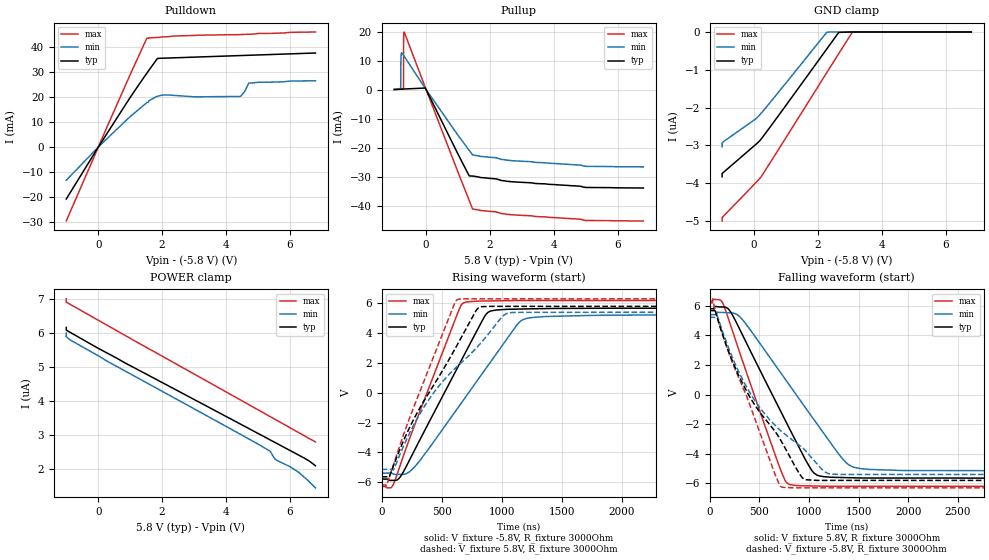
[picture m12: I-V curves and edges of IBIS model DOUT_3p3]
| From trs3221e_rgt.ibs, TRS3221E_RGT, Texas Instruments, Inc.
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[Model]   DOUT_3p3
Model_type   3-state
Polarity   Inverting
Vmeas = 1.65
Vref = 0
Cref = 150pF
Rref = 3000
|variable   typ   min   max
C_comp   6.67pF   5.86pF   7.62pF
|C_pullup   6.73pF   5.94pF   7.44pF
|C_pulldown   6.54pF   5.54pF   7.65pF
[Voltage Range]   11.6   10.8   12.6
[Temperature Range]   27   110   -40
[Pullup Reference]   5.8   5.4   6.3
[Pulldown Reference]   -5.8   -5.4   -6.3
[Power Clamp Reference]   5.8   5.4   6.3
[GND Clamp Reference]   -5.8   -5.4   -6.3
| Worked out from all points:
|   slope of the pulldown table from 0 to 1.74 V, typ, clamps not added: 52 ohm
|   slope of the pullup table from 0 to 1.74 V, typ, clamps not added: 57.4 ohm
|   falling waveform, V_fixture 5.8V, R_fixture 3000Ohm: 20-80 % time 516ns typ, 670ns min, 385ns max; typ from 5.8 V to -5.64 V
|   rising waveform, V_fixture -5.8V, R_fixture 3000Ohm: 20-80 % time 446ns typ, 563ns min, 354ns max; typ from -5.8 V to 5.67 V
|   rising waveform, V_fixture 5.8V, R_fixture 3000Ohm: 20-80 % time 475ns typ, 608ns min, 355ns max; typ from -5.64 V to 5.8 V
|   falling waveform, V_fixture -5.8V, R_fixture 3000Ohm: 20-80 % time 586ns typ, 680ns min, 425ns max; typ from 5.67 V to -5.8 V
[Pulldown]
|   Voltage   I(typ)   I(min)   I(max)
-1V       -20.69mA   -13.21mA   -29.48mA
121.7mV   2.419mA    1.551mA    3.562mA
975.3mV   19.36mA    11.94mA    28.26mA
1.525V    29.58mA    17.81mA    43.51mA
1.856V    35.45mA    20.31mA    43.81mA
2.156V    35.58mA    20.85mA    44.08mA
3.033V    35.96mA    20.07mA    44.64mA
4.428V    36.57mA    20.23mA    44.94mA
4.464V    36.58mA    20.4mA     44.96mA
4.586V    36.64mA    22.27mA    45.02mA
4.713V    36.69mA    25.62mA    45.08mA
6.8V      37.6mA     26.51mA    45.97mA
[GND Clamp]
|   Voltage   I(typ)   I(min)   I(max)
-1V       -3.829uA   -3.033uA   -4.999uA
-1V       -3.77uA    -2.976uA   -4.939uA
-1V       -3.759uA   -2.965uA   -4.928uA
-1V       -3.742uA   -2.949uA   -4.912uA
-999.7mV  -3.742uA   -2.934uA   -4.909uA
-947.7mV  -3.704uA   -2.894uA   -4.86uA
29.67mV   -2.991uA   -2.31uA    -4.007uA
240.5mV   -2.811uA   -2.129uA   -3.804uA
2.272V    -452.5nA   -9.865nA   -1.078uA
2.65V     -10.91nA   0A         -571.9nA
3.071V    0A         0A         -11.58nA
6.8V      0A         0A         0A
[Pullup]
|   Voltage   I(typ)   I(min)   I(max)
-1V       58.5uA     47.9uA     71.7uA
-800mV    163.2uA    219.8uA    162.4uA
-787.3mV  169.9uA    11.17mA    168.1uA
-778.7mV  174.4uA    12.51mA    172.1uA
-709.6mV  210.6uA    11.87mA    203.4uA
-706.5mV  212.2uA    11.82mA    1.796mA
-705.2mV  212.9uA    11.8mA     14.41mA
-703.4mV  213.9uA    11.77mA    18.21mA
-686.7mV  222.6uA    11.49mA    19.85mA
-24.92mV  569.4uA    410.9uA    731.3uA
1.455V    -29.77mA   -22.5mA    -41.14mA
6.8V      -33.87mA   -26.6mA    -45.24mA
[POWER Clamp]
|   Voltage   I(typ)   I(min)   I(max)
-1V       6.156uA    5.99uA     6.993uA
-1V       6.096uA    5.932uA    6.931uA
-1V       6.077uA    5.912uA    6.913uA
-999.8mV  6.077uA    5.883uA    6.897uA
-868.1mV  6.007uA    5.785uA    6.827uA
970.8mV   5.052uA    4.814uA    5.854uA
5.366V    2.871uA    2.54uA     3.554uA
5.514V    2.798uA    2.325uA    3.476uA
5.566V    2.772uA    2.277uA    3.449uA
6V        2.555uA    2.08uA     3.221uA
6.25V     2.431uA    1.93uA     3.09uA
6.8V      2.106uA    1.459uA    2.802uA
[Ramp]
R_load = 3000
|   typ   min   max
dV/dt_r   6.88152/4.46257e-07   6.37012/5.61965e-07   7.49789/3.54595e-07
dV/dt_f   6.86701/5.15292e-07   6.32828/6.69404e-07   7.49815/3.85293e-07
[Falling Waveform]
V_fixture = 5.8V
V_fixture_min = 5.4V
V_fixture_max = 6.3V
R_fixture = 3000Ohm
C_fixture = 0F
|   Time   V(typ)   V(min)   V(max)
0s        5.8V       5.4V       6.3V
136.4ns   5.912V     5.54V      6.107V
209.2ns   5.601V     5.519V     4.713V
317.9ns   4.199V     5.153V     2.525V
693.4ns   -842.9mV   1.677V     -4.712V
794.9ns   -2.189V    714.4mV    -6.045V
1.051us   -5.31V     -1.711V    -6.174V
1.327us   -5.601V    -4.254V    -6.191V
1.469us   -5.625V    -4.937V    -6.191V
4us       -5.645V    -5.148V    -6.197V
[Rising Waveform]
V_fixture = -5.8V
V_fixture_min = -5.4V
V_fixture_max = -6.3V
R_fixture = 3000Ohm
C_fixture = 0F
|   Time   V(typ)   V(min)   V(max)
0s        -5.8V      -5.399V    -6.3V
86.73ns   -5.887V    -5.416V    -6.303V
166ns     -5.511V    -5.479V    -4.578V
293.7ns   -3.543V    -4.798V    -1.769V
647.4ns   1.918V     -875mV     5.625V
688.6ns   2.551V     -409.7mV   6.054V
887.3ns   5.401V     1.837V     6.16V
1.13us    5.612V     4.575V     6.185V
1.213us   5.625V     4.995V     6.188V
4us       5.67V      5.217V     6.197V
[Rising Waveform]
V_fixture = 5.8V
V_fixture_min = 5.4V
V_fixture_max = 6.3V
R_fixture = 3000Ohm
C_fixture = 0F
|   Time   V(typ)   V(min)   V(max)
0s        -5.645V    -5.148V    -6.197V
40.78ns   -5.644V    -5.147V    -6.219V
62.79ns   -5.663V    -5.146V    -5.677V
99.89ns   -4.844V    -5.153V    -4.799V
346.4ns   -627.5mV   -1.038V    662.7mV
635.1ns   3.293V     1.807V     6.263V
807.3ns   5.694V     3.164V     6.298V
1.008us   5.797V     5.133V     6.298V
1.085us   5.797V     5.384V     6.298V
4us       5.8V       5.4V       6.3V
[Falling Waveform]
|Gnd
V_fixture = -5.8V
V_fixture_min = -5.4V
V_fixture_max = -6.3V
R_fixture = 3000Ohm
C_fixture = 0F
|   Time   V(typ)   V(min)   V(max)
0s        5.67V      5.217V     6.197V
31.26ns   5.667V     5.216V     6.344V
76.53ns   5.193V     5.336V     5.247V
209.2ns   2.586V     2.828V     2.506V
346.4ns   567.5mV    824.4mV    296mV
526.1ns   -1.377V    -1.072V    -2.949V
726.4ns   -3.214V    -2.503V    -6.251V
932.1ns   -5.617V    -3.571V    -6.298V
1.237us   -5.797V    -5.381V    -6.298V
4us       -5.8V      -5.399V    -6.3V
